(* Logix 5000 DataType export Seq_Type; software revision 20.05 *)

TYPE Seq_Type :   // Sequence Information
STRUCT
   Step_Num : DINT;   // Current step number
   Running : BOOL;   // Running indication
   PC_Start : BOOL;   // Sequence start request from PC
   LTP_Start : BOOL;   // Sequence start request from LTP
   Ons : BOOL;   // One-shot storage to start
   Auto_Start : BOOL;   // Auto-start request
   Auto_Ons : BOOL;   // Auto-start one-shot storage
   Req_Tmr : TIMER;   // Auto-start hold timer
END_STRUCT
END_TYPE
